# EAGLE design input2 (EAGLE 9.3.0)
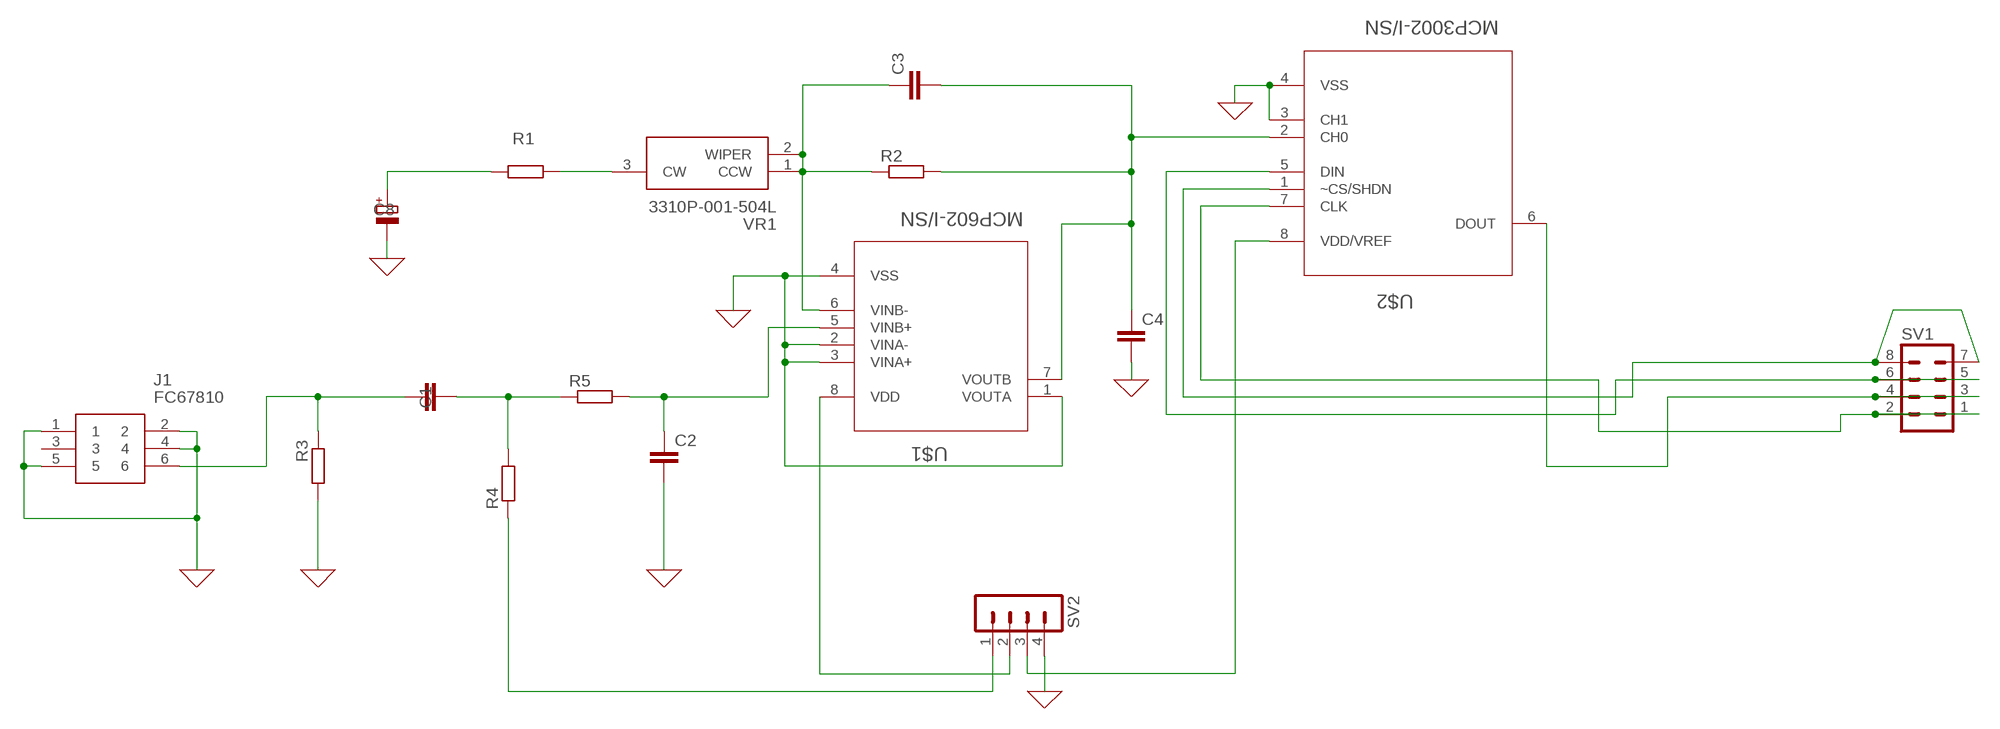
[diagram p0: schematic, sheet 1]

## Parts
C1  C-EUC0805  [C0805]
C2  C-EUC0805  [C0805]
C3  C-EUC0805  [C0805]
C4  C-EUC0805  [C0805]
C8  CPOL-EUE2-5  [E2-5]
J1  FC67810  [FC67810]
R1  R-EU_R0805  [R0805]
R2  R-EU_R0805  [R0805]
R3  R-EU_R0805  [R0805]
R4  R-EU_R0805  [R0805]
R5  R-EU_R0805  [R0805]
SV1  MA04-2  [MA04-2]
SV2  MA04-1  [MA04-1]
U$1  MCP602-I/SN  [SOIC127P600X175-8N]
U$2  MCP3002-I/SN  [SOIC127P600X175-8N]
VR1  3310P-001-504L  [3310P-1]

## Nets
0: C2.2 C4.2 C8.- J1.1 J1.2 J1.4 J1.5 R3.2 SV2.4 U$1.1(VOUTA) U$1.2(VINA-) U$1.3(VINA+) U$1.4(VSS) U$2.3(CH1) U$2.4(VSS) ; supply symbol labelled GND
N$1: SV1.5 SV1.6 U$2.5(DIN)
N$3: C1.2 R4.2 R5.1
N$4: C2.1 R5.2 U$1.5(VINB+)
N$5: C3.2 C4.1 R2.2 U$1.7(VOUTB) U$2.2(CH0)
N$6: SV1.7 SV1.8 U$2.1(~CS/SHDN)
N$7: C3.1 R2.1 U$1.6(VINB-) VR1.1(CCW) VR1.2(WIPER)
N$8: R1.1 VR1.3(CW)
N$9: C8.+ R1.2
N$10: SV1.1 SV1.2 U$2.7(CLK)
N$11: SV1.3 SV1.4 U$2.6(DOUT)
N$12: SV2.2 U$1.8(VDD)
N$13: R4.1 SV2.1
N$14: SV2.3 U$2.8(VDD/VREF)
N$15: C1.1 J1.6 R3.1
Unconnected: J1.3

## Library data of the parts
C1-C4 = rcl:C-EU: CAPACITOR, European symbol; SPICEPREFIX: C
C8 = rcl:CPOL-EU: POLARIZED CAPACITOR, European symbol; SPICEPREFIX: C
J1 = SamacSys_Parts:FC67810: S1K,Sealed jack sockets, stereo 1/4" Cliff Electronics 6.35mm PCB Mount Stereo Jack Socket, 5A Source: Datasheet; DESCRIPTION: S1K,Sealed jack sockets, stereo 1/4" Cliff Electronics 6.35mm PCB Mount Stereo Jack Socket, 5A; HEIGHT: mm; MANUFACTURER_NAME: CLIFF ELECTRONIC COMPONENTS; MANUFACTURER_PART_NUMBER: FC67810; MOUSER_PART_NUMBER: 8051646; MOUSER_PRICE-STOCK: http://uk.rs-online.com/web/p/products/8051646; RS_PART_NUMBER: 8051646; RS_PRICE-STOCK: http://uk.rs-online.com/web/p/products/8051646
R1-R5 = rcl:R-EU_: RESISTOR, European symbol; SPICEPREFIX: R
SV1 = con-lstb:MA04-2: PIN HEADER; OC_FARNELL: unknown; OC_NEWARK: unknown
SV2 = con-lstb:MA04-1: PIN HEADER; OC_FARNELL: unknown; OC_NEWARK: unknown
U$1 = Microchip_By_element14_Batch_1:MCP602-I/SN: CMOS Op Amp; MPN: MCP602-I/SN; OC_FARNELL: 9758666; OC_NEWARK: 12C1813;; PACKAGE: SOIC-8; SUPPLIER: Microchip
U$2 = Microchip_By_element14_Batch_1:MCP3002-I/SN: Dual Channel 10-Bit A/D Converter; DESCRIPTION: Dual Channel 10-Bit A/D Converter; MPN: MCP3002-I/SN; OC_FARNELL: 1834969; OC_NEWARK: 59K0225; PACKAGE: SOIC-8; SUPPLIER: Microchip
VR1 = SamacSys_Parts:3310P-001-504L: Bourns Audio Potentiometer 3310P-001 Series with a 3.17 mm Dia. Shaft 500k +/-20% 0.25W +/-1000ppm/C, Linear Source: Datasheet; DESCRIPTION: Bourns Audio Potentiometer 3310P-001 Series with a 3.17 mm Dia. Shaft 500k +/-20% 0.25W +/-1000ppm/C, Linear; HEIGHT: mm; MANUFACTURER_NAME: Bourns; MANUFACTURER_PART_NUMBER: 3310P-001-504L; RS_PART_NUMBER: 6916917

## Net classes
0 default: width 0.305 mm, drill 0.762 mm, clearance 0.508 mm

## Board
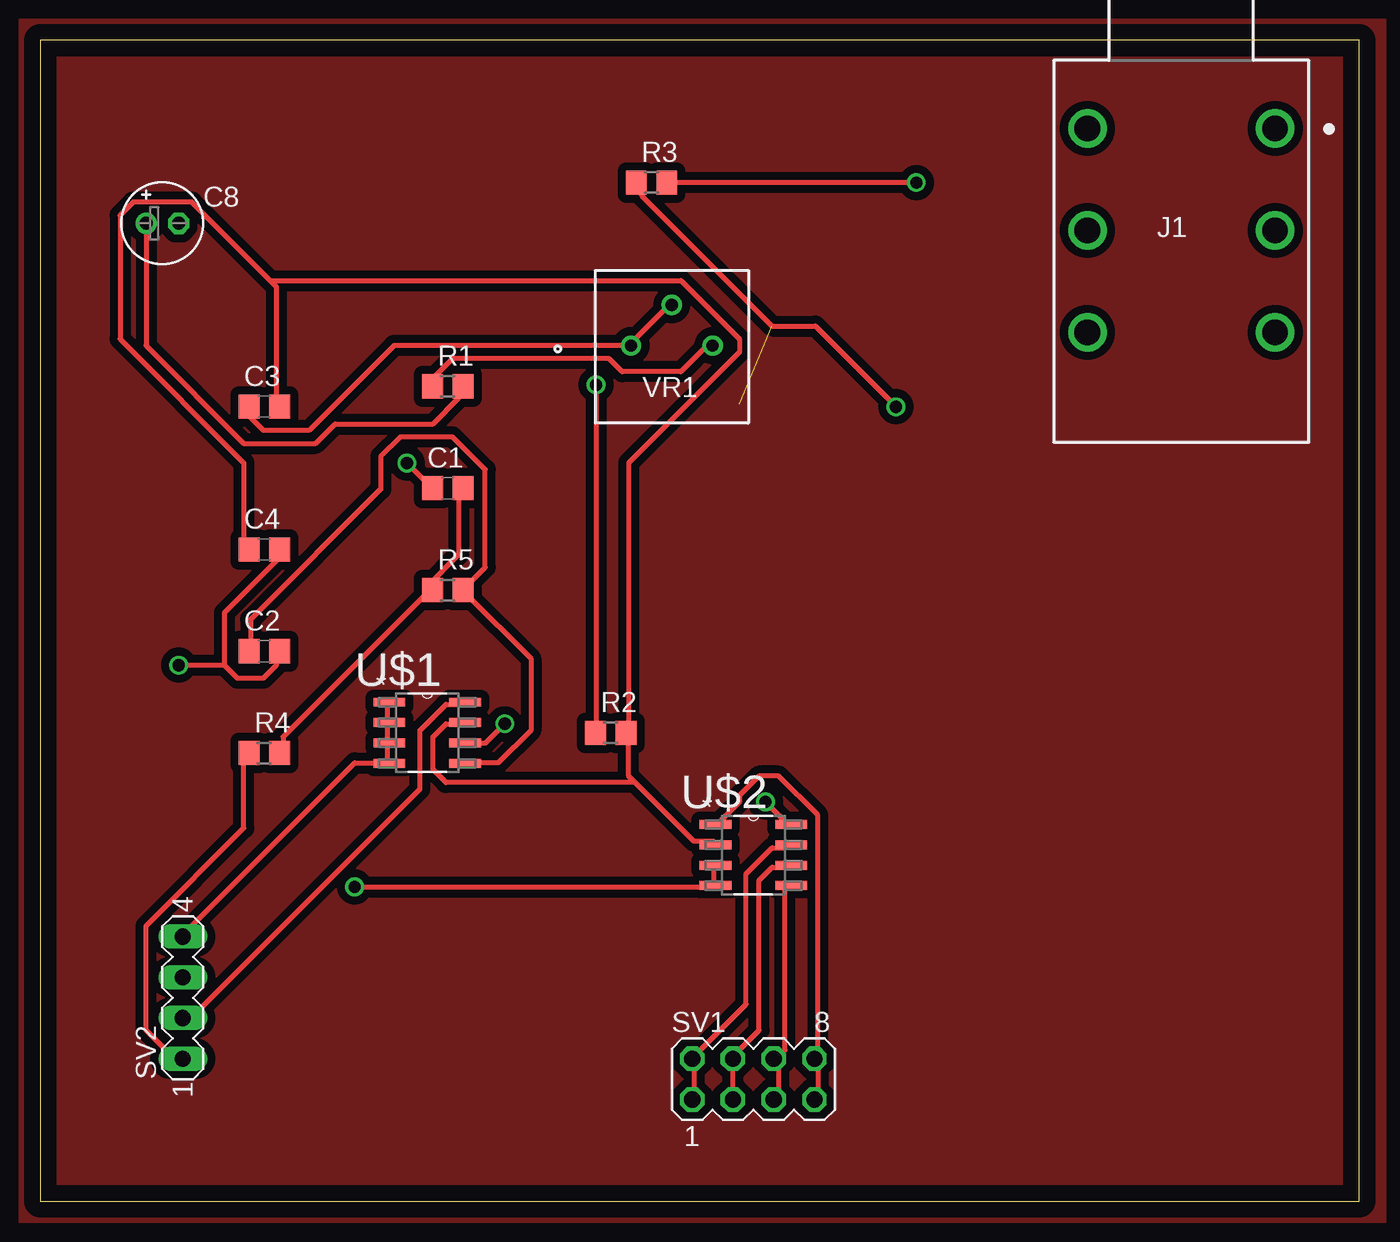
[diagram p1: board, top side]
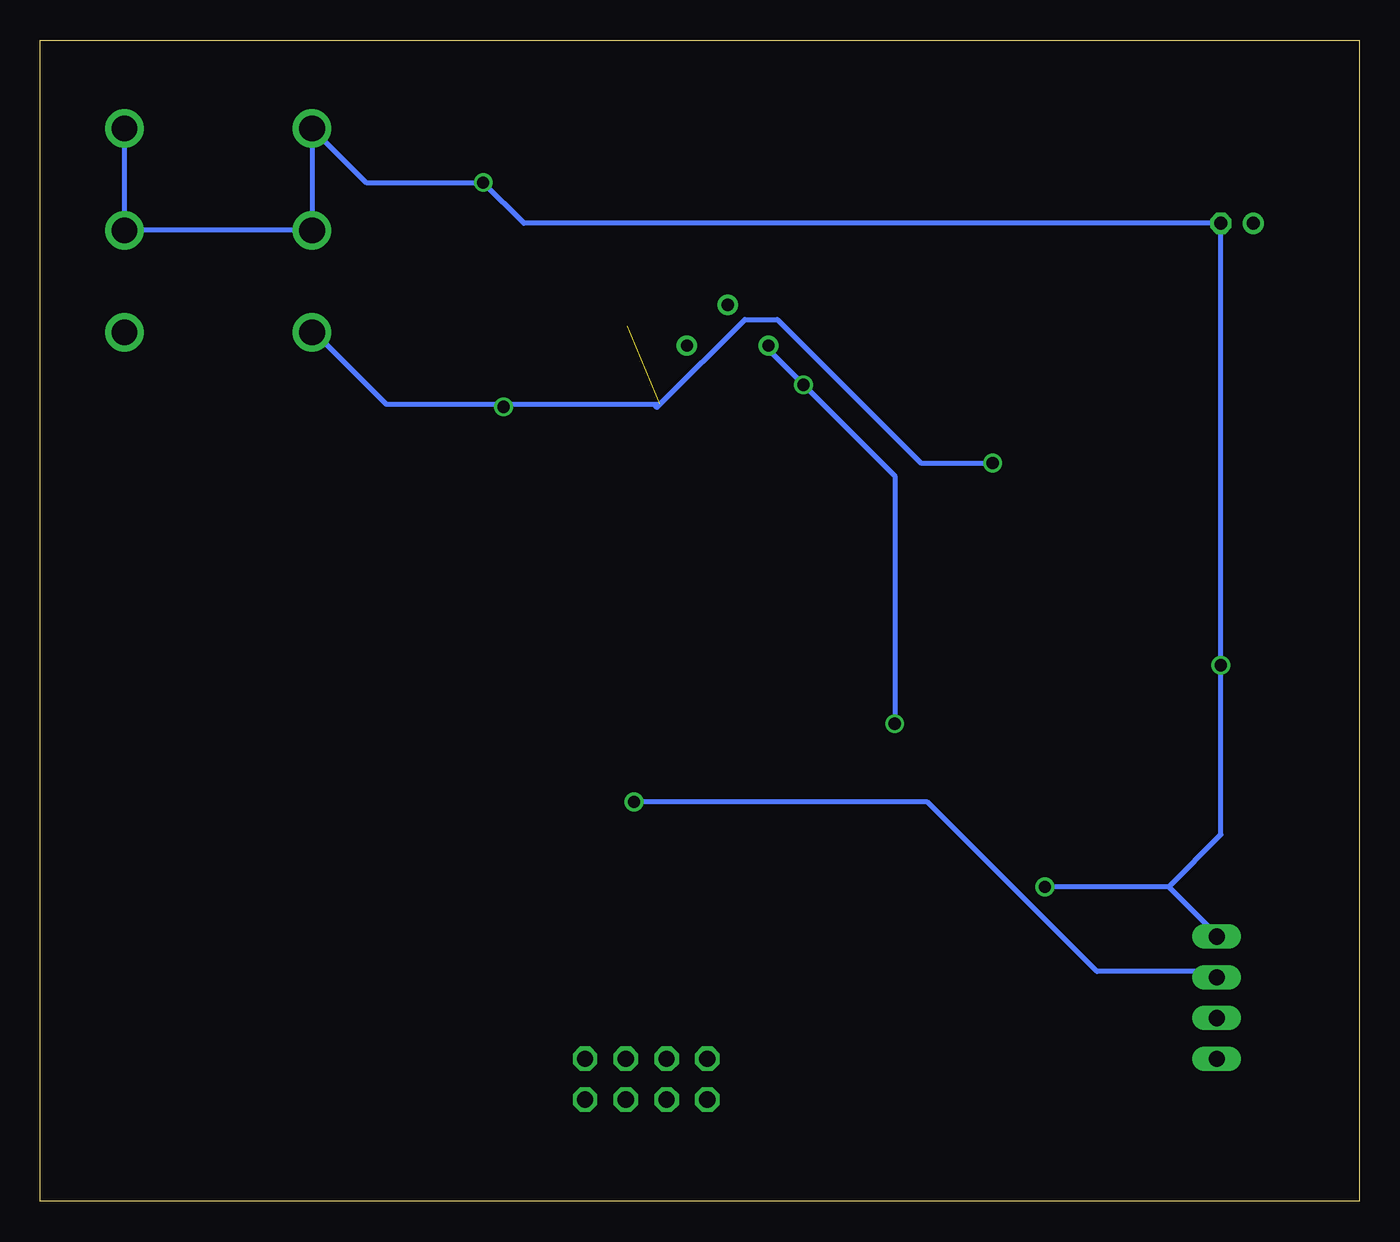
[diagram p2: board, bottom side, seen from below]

Size 82.22 x 72.38 mm. Coordinates in mm from the lower left corner, seen from the top.
Outline: 0,0 82.22,0 82.22,72.38 0,72.38 0,0
Copper layers (1*16): Top 0.035mm / dielectric 1.5mm / Bottom 0.035mm
Design rules "default": minimum track width 6mil, minimum drill 0.35mm, track to track 6mil, track to pad 6mil, pad to pad 6mil, via to via 6mil, smd to smd 6mil, copper to edge 40mil, drill to drill 6mil, minimum pad ring 10mil, minimum via ring 8mil, stop-mask expansion 4mil, vias tented up to drill 0mil, thermal gap 10mil

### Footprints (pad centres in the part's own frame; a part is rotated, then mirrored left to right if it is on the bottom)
C0805 = smd 1.3 x 1.5: 1 -0.95,0; 2 0.95,0
E2-5 = drill 0.813 pad 1.27: + -1.016,0 | drill 0.813 pad 1.27 octagon: - 1.016,0
FC67810 = drill 1.6 pad 2.4: 1 5.85,-4.25; 2 5.85,-10.6; 3 5.85,-16.95; 4 -5.85,-4.25; 5 -5.85,-10.6; 6 -5.85,-16.95
R0805 = smd 1.3 x 1.5: 1 -0.95,0; 2 0.95,0
MA04-2 = drill 1.016 octagon: 1 -3.81,-1.27; 2 -3.81,1.27; 3 -1.27,-1.27; 4 -1.27,1.27; 5 1.27,-1.27; 6 1.27,1.27; 7 3.81,-1.27; 8 3.81,1.27
MA04-1 = drill 1.016 long: 1 -3.81,0; 2 -1.27,0; 3 1.27,0; 4 3.81,0
SOIC127P600X175-8N = smd 1.981 x 0.559: 1 -2.362,1.905; 2 -2.362,0.635; 3 -2.362,-0.635; 4 -2.362,-1.905; 5 2.362,-1.905; 6 2.362,-0.635; 7 2.362,0.635; 8 2.362,1.905
3310P-1 = drill 0.76 pad 1.26: 1 -2.54,0; 2 0,2.54; 3 2.54,0

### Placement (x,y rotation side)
C1  25.4,44.45 0 top
C2  13.97,34.29 0 top
C3  13.97,49.53 0 top
C4  13.97,40.64 0 top
C8  7.62,60.96 0 top
J1  71.12,71.12 0 top
R1  25.4,50.8 0 top
R2  35.56,29.21 0 top
R3  38.1,63.5 0 top
R4  13.97,27.94 0 top
R5  25.4,38.1 0 top
SV1  44.45,7.62 0 top
SV2  8.89,12.7 90 top
U$1  24.13,29.21 0 top
U$2  44.45,21.59 0 top
VR1  39.37,53.34 0 top

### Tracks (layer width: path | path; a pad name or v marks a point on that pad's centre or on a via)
0  (via drill 0.75, 0.76)
  Top 0.305: 77.32,60.66 J1.2 76.91,60.66 | 77.32,66.75 J1.1 | v54.61,63.5 R3.2 | 65.13,60.66 J1.5 65.53,60.66 | 65.13,66.75 J1.4 | 11.48,33.43 12.29,32.61 13.92,32.61 14.73,33.43 14.73,34.24 C2.2 | 11.48,33.43 11.48,36.68 15.14,40.34 C4.2 | 21.64,28.55 21.64,27.33 | 21.64,29.77 21.64,30.99 U$1.1 | 21.64,29.77 21.64,28.55 | 21.64,28.55 U$1.3 | 21.64,29.77 U$1.2 | 41.96,19.61 41.96,20.83 U$2.3 | v19.61,19.61 41.96,19.61 | 41.96,19.61 U$2.4 | 21.64,27.33 19.61,27.33 9.04,16.76 SV2.4 | 21.64,27.33 U$1.4 | v8.64,33.43 11.48,33.43
  Bottom 0.305: 11.89,19.61 v19.61,19.61 | 11.89,19.61 9.04,16.76 SV2.4 | 11.89,19.61 8.64,22.86 v8.64,33.43 C8.- 52.07,60.96 | 65.13,60.66 J1.5 | 52.12,61.06 52.07,60.96 | J1.5 76.2,60.52 | 76.2,60.52 J1.2 | J1.1 76.97,61.29 76.2,60.52 | J1.5 J1.4 61.9,63.5 v54.61,63.5 52.07,60.96
GND
  pour Top: -1.27,73.66 -1.27,-1.27 83.82,-1.27 83.82,73.66
N$1
  Top 0.305: U$2.5 46.43,19.61 46.43,9.45 46.02,9.04 SV1.6 46.02,8.64 46.02,6.6 SV1.5
N$3
  Top 0.305: R4.2 15.14,28.14 15.14,28.96 24.08,37.9 R5.1 24.08,38.3 26.11,40.34 26.11,44.4 C1.2
N$4
  Top 0.305: C2.1 13.11,34.65 13.11,36.27 21.23,44.4 21.23,46.43 22.45,47.65 25.7,47.65 27.74,45.62 27.74,39.52 26.52,38.3 R5.2 26.52,37.9 30.58,33.83 30.58,29.36 28.55,27.33 26.52,27.33 U$1.5
N$5
  Top 0.305: 37.08,26.11 40.74,22.45 41.96,22.45 U$2.2 | 37.08,26.11 36.68,26.52 36.68,28.96 R2.2 36.68,29.36 36.68,46.03 43.59,52.93 43.59,53.75 39.93,57.4 14.33,57.4 | 37.08,26.11 25.3,26.11 24.49,26.92 24.49,28.96 25.3,29.77 26.11,29.77 U$1.7 | 14.33,57.4 14.73,57 14.73,49.68 C3.2 | 14.33,57.4 9.45,62.28 5.79,62.28 4.98,61.47 4.98,53.75 12.7,46.03 12.7,40.74 C4.1
N$6
  Top 0.305: U$2.1 42.37,23.67 43.59,24.89 43.59,25.3 44.81,26.52 46.02,26.52 48.46,24.08 48.46,9.04 SV1.8 48.46,8.64 48.46,6.6 SV1.7
N$7  (via drill 0.76)
  Top 0.305: 36.68,53.34 22.05,53.34 16.76,48.06 13.92,48.06 13.11,48.87 13.11,49.28 C3.1 | v34.65,50.9 34.65,29.36 R2.1 | v28.96,29.77 27.74,28.55 26.52,28.55 U$1.6 | 36.68,53.34 39.12,55.78 VR1.2 | 36.68,53.34 VR1.1
  Bottom 0.305: VR1.1 37.08,53.34 v34.65,50.9 28.96,45.21 v28.96,29.77
N$8
  Top 0.305: R1.1 24.49,50.9 24.49,51.31 25.7,52.53 35.46,52.53 36.27,51.71 39.93,51.71 41.55,53.34 VR1.3
N$9
  Top 0.305: C8.+ 6.6,53.34 12.7,47.24 17.17,47.24 18.39,48.46 24.49,48.46 26.11,50.09 26.11,50.5 R1.2
N$10
  Top 0.305: U$2.7 46.43,22.05 45.62,22.05 43.99,20.42 43.99,12.29 40.74,9.04 SV1.2 40.74,8.64 40.74,6.6 SV1.1
N$11
  Top 0.305: U$2.6 46.43,20.83 45.62,20.83 44.81,20.02 44.81,10.67 43.18,9.04 SV1.4 SV1.3
N$12
  Top 0.305: U$1.8 26.11,30.99 25.3,30.99 23.67,29.36 23.67,25.71 9.04,11.07 SV2.2
N$13
  Top 0.305: R4.1 12.7,27.74 12.7,23.27 6.6,17.17 6.6,10.67 8.64,8.64 SV2.1
N$14  (via drill 0.76)
  Top 0.305: v45.21,24.89 46.43,23.67 U$2.8
  Bottom 0.305: v45.21,24.89 26.92,24.89 16.36,14.33 9.04,14.33 SV2.3
N$15  (via drill 0.76)  (1 unrouted)
  Top 0.305: v22.86,46.03 24.08,44.81 C1.1 | R3.1 37.49,63.5 37.49,62.69 45.62,54.56 48.31,54.56 v53.34,49.53 | 65.13,54.56 J1.6
  Bottom 0.305: v22.86,46.03 27.33,46.03 36.27,54.97 38.3,54.97 43.59,49.68 | 43.59,49.68 43.79,49.48 arc-90 43.84,49.53 | 43.59,49.68 60.66,49.68 65.13,54.15 J1.6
